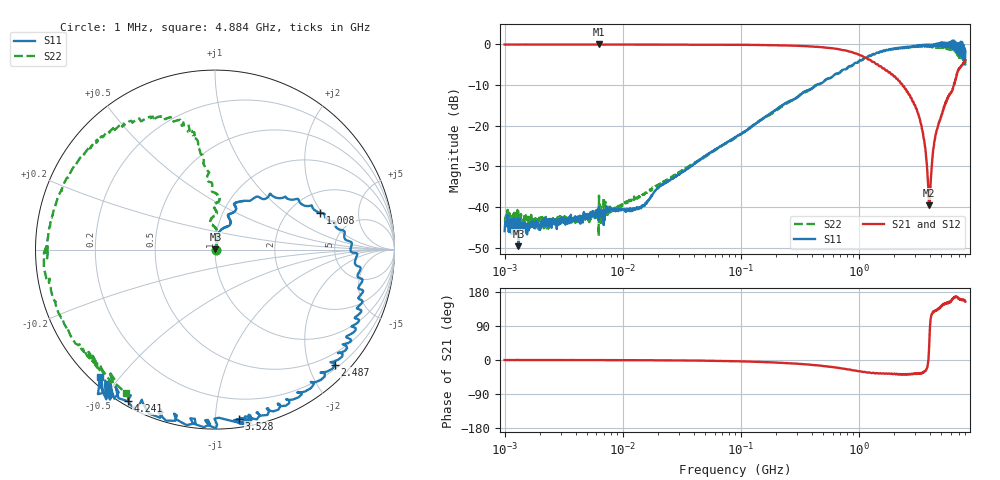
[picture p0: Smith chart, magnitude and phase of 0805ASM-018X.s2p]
!s-Parameter Generated by FASTRON Sdn. Bhd.
!FASTRON P/N : 0805ASM-018X
!Keysight Technologies: E5071C_MY46733604_B.14.02
!Date: Fri Jun 19 14:47:51 2026
!Version  :Rev00  Fri Jun 19 14:47:51 2026
!Data & Calibration Information:
!Freq  S11:SOLT2(ON)  S21:SOLT2(ON)  S12:SOLT2(ON)  S22:SOLT2(ON)
!PortZ  Port1:50+j0  Port2:50+j0
!When reading reference impedance value at option line is always used.
! Remarks : This data is being provided solely for informational purposes.
# Hz S dB R 50
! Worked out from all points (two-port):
!   1601 points, 1 MHz to 8 GHz, reference 50 ohm
!   highest |S21| = -0.02 dB at 6.301 MHz (marker M1); lowest = -39.6 dB at 3.953 GHz (marker M2)
!   |S21| within 3 dB of the highest: start of sweep to 1.086 GHz
!   lowest |S11| = -49.6 dB at 1.31 MHz (marker M3), VSWR 1.01, Z = 50.2 + j0.221 ohm
!   |S11| at or under -10 dB: start of sweep to 437 MHz
!   |S22| runs from -47.1 to -0.4 dB; largest |S21 - S12| = 0.023
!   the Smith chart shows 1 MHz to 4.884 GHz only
!   S11 on the Smith chart (normalised r, x): 1 MHz: 1.01, -0.00; 1.008 GHz: 2.88, +1.93; 2.487 GHz: 0.27, -2.46; 3.528 GHz: 0.06, -1.15; 4.241 GHz: 0.02, -0.58; 4.884 GHz: 0.03, -0.44
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1000000  -45.90 -7.4  -0.07 -0.1  -0.06 -0.1  -43.30 0.8
1310238  -49.60 41.7  -0.09 0.1  -0.07 -0.2  -40.80 -15.0
4479405  -43.00 24.4  -0.07 -0.2  -0.07 -0.2  -43.10 28.3
6301378  -39.90 33.5  -0.01 -0.5  -0.02 -0.3  -37.20 38.7
1.414737e7  -39.90 59.5  -0.06 -0.6  -0.08 -0.6  -37.20 52.9
2.00676e7  -35.10 62.6  -0.07 -0.8  -0.08 -0.7  -34.50 66.3
8.994653e7  -22.80 76.5  -0.11 -3.2  -0.12 -3.2  -23.00 81.2
4.006501e8  -10.90 66.0  -0.54 -12.9  -0.55 -12.9  -10.70 85.2
1.007883e9  -4.12 19.3  -2.63 -29.7  -2.64 -29.8  -4.05 99.8
1.7949e9  -1.28 -19.0  -6.94 -35.6  -6.94 -35.9  -1.30 125.0
2.486897e9  -0.66 -43.9  -11.00 -36.9  -11.10 -37.2  -0.83 146.0
3.122398e9  -0.56 -75.7  -16.40 -36.9  -16.50 -36.5  -0.60 176.0
3.527775e9  -0.42 -81.9  -22.80 -33.3  -22.70 -33.0  -0.61 -179.0
3.95342e9  -0.19 -103.0  -39.60 44.8  -39.60 44.6  -0.60 -156.0
4.075033e9  -0.13 -112.0  -33.30 110.0  -33.30 110.0  -0.56 -149.0
4.240668e9  -0.22 -120.0  -26.80 127.0  -26.80 126.0  -0.73 -143.0
4.88448e9  -0.40 -132.0  -18.60 137.0  -18.60 138.0  -0.54 -122.0
5.472309e9  -0.56 -155.0  -14.30 148.0  -14.30 148.0  -0.78 -78.7
5.918038e9  0.55 -156.0  -12.20 154.0  -12.10 154.0  -1.07 -74.5
6.534915e9  0.14 -163.0  -8.95 167.0  -8.97 166.0  -1.12 -27.0
7.306013e9  0.65 165.0  -5.45 160.0  -5.32 160.0  -2.53 -11.4
8e9  -1.62 133.0  -3.81 154.0  -3.71 154.0  -3.79 28.5
